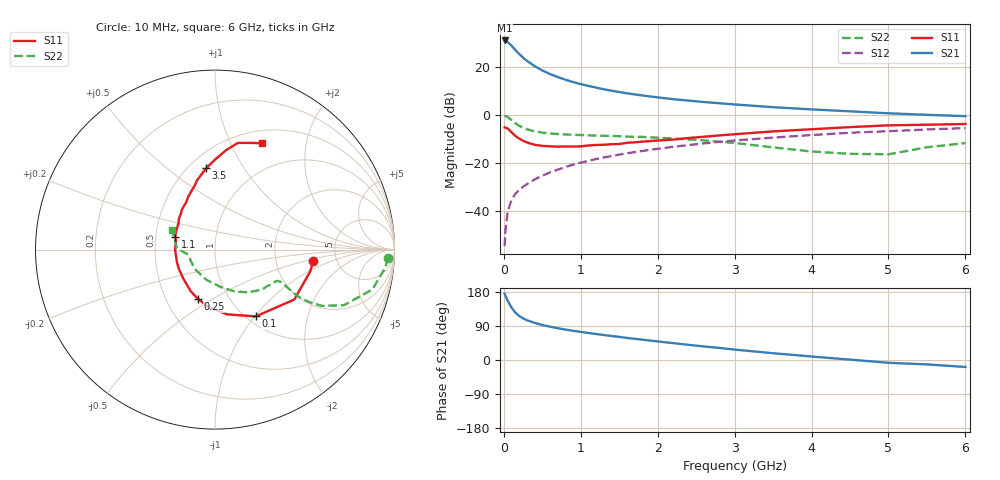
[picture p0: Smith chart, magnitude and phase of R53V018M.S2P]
! SIEMENS Small Signal Semiconductors
! BFR183
! Si NPN RF Bipolar Junction Transistor in SOT23
! VCE = 3 V  IC = 18 mA
! Common Emitter S-Parameters:  May  1996
# GHz  S  MA  R  50
!  f  S11  S21  S12  S22
! GHz  MAG  ANG  MAG  ANG  MAG  ANG  MAG  ANG
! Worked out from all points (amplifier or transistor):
!   36 points, 10 MHz to 6 GHz, reference 50 ohm
!   highest |S21| = 30.9 dB at 10 MHz (marker M1)
!   |S21| within 3 dB of that: start of sweep to 123 MHz
!   unconditionally stable (mu >= 1): 579.7 MHz to 2.392 GHz
!   at 250 MHz: K = 0.79, MSG = 26.8 dB, |S12| = -29.8 dB
!   at 1.4 GHz: K = 1.05, MAG = 12.2 dB, |S12| = -17.1 dB
!   at 6 GHz: K = 0.90, MSG = 2.5 dB, |S12| = -5.5 dB
!   S11 on the Smith chart (normalised r, x): 10 MHz: 3.32, -0.63; 100 MHz: 1.10, -1.01; 250 MHz: 0.72, -0.43; 1.1 GHz: 0.63, +0.10; 3.5 GHz: 0.61, +0.69; 6 GHz: 0.65, +1.32
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0.01  0.5512 -6.9  35 174.9  0.0019 90.7  0.9657 -2.7
0.02  0.5441 -13.0  34.67 169.7  0.004 83.8  0.9548 -5.9
0.05  0.5222 -32.2  32.61 156.3  0.0099 78.6  0.905 -14.2
0.1  0.4359 -58.6  27.24 138.2  0.0173 71.2  0.7827 -23.3
0.15  0.367 -79.5  22.17 124.9  0.0233 67.4  0.6725 -27.8
0.2  0.323 -96.1  18.31 116.2  0.0276 66.8  0.5963 -29.2
0.25  0.2899 -109.2  15.4 109.8  0.0324 67.0  0.5408 -29.4
0.3  0.2688 -120.1  13.24 104.9  0.0367 68.1  0.5034 -29.0
0.4  0.24 -136.8  10.3 98.2  0.0458 69.1  0.4575 -27.7
0.5  0.2285 -151.4  8.35 92.3  0.0549 70.2  0.4298 -26.7
0.6  0.2236 -161.4  7.057 87.9  0.0643 70.4  0.4134 -26.2
0.7  0.22 -170.6  6.116 83.9  0.0733 70.8  0.402 -26.2
0.8  0.222 -178.3  5.369 80.3  0.083 70.1  0.3933 -26.4
0.9  0.2216 174.8  4.8 77.1  0.0929 70.1  0.3872 -26.7
1.1  0.2329 162.0  3.996 71.4  0.1118 69.0  0.3779 -28.7
1.3  0.2404 152.2  3.404 65.9  0.1314 67.3  0.3691 -30.5
1.6  0.2641 139.8  2.81 58.2  0.1602 64.8  0.3551 -34.8
2.2  0.3075 121.6  2.122 44.5  0.2182 58.6  0.3259 -44.9
3.5  0.456 96.3  1.446 17.9  0.3389 42.4  0.2123 -80.8
4.5  0.5588 83.5  1.188 1.0  0.4271 29.8  0.1561 -137.3
5.5  0.6264 71.6  1.005 -11.6  0.4994 18.0  0.2132 178.0
6  0.6481 66.2  0.942 -18.4  0.5332 10.3  0.2609 155.8
